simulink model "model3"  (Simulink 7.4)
settings: Solver=ode4  SolverMode=SingleTasking  StartTime=0.0  StopTime=10  FixedStep=1e-3  RelTol=1e-3
libraries: simulink x2

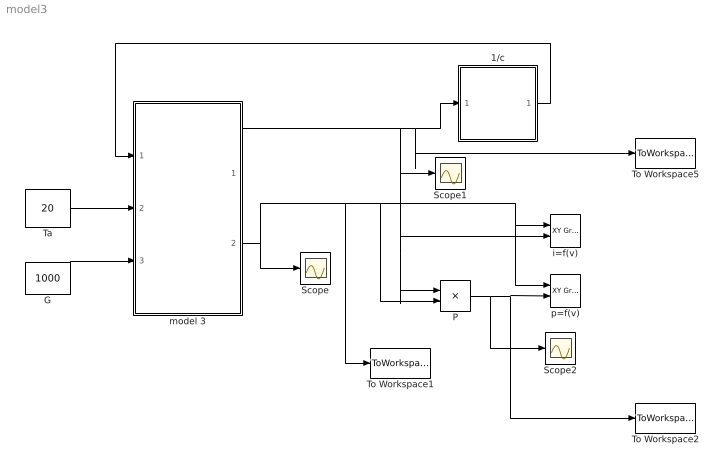
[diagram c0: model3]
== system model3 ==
  1/c : Subsystem
  G : Constant  Value=1000  OutDataType=sfix(16)  OutScaling=2^0
  P : Product  OutDataType=sfix(16)  OutScaling=2^0
  Scope : Scope
  Scope1 : Scope
  Scope2 : Scope
  Ta : Constant  Value=20  OutDataType=sfix(16)  OutScaling=2^0
  To Workspace1 : ToWorkspace  VariableName=v  SampleTime=-1  SaveFormat=Array
  To Workspace2 : ToWorkspace  VariableName=p  SampleTime=-1  SaveFormat=Array
  To Workspace5 : ToWorkspace  VariableName=i  SampleTime=-1  SaveFormat=Array
  i=f(v) : simulink/Sinks/XY Graph  SystemSampleTime=-1  xmin=0  xmax=50  ymin=0  ymax=5  st=-1
  model 3 : Subsystem  mask{beta_ref=-152e-3, alpha_ref=1.4e-3, Vm=35, Im=3.15, Voc=43.5, Isc=3.45, Tjref=25, Esref=1000, Noct=45}
  p=f(v) : simulink/Sinks/XY Graph  SystemSampleTime=-1  xmin=0  xmax=50  ymin=0  ymax=150  st=-1
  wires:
  1/c/1(Vdc) -> model 3/1(v)
  model 3/1(i+di) -> Scope1/1, P/1, i=f(v)/2, 1/c/1(Idc), To Workspace5/1
  P/1 -> Scope2/1, p=f(v)/2, To Workspace2/1
  model 3/2(v+dv1) -> Scope/1, i=f(v)/1, p=f(v)/1, P/2, To Workspace1/1
  Ta/1 -> model 3/2(Ta)
  G/1 -> model 3/3(G)

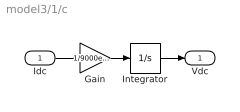
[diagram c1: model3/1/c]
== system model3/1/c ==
  Idc : Inport  OutDataType=sfix(16)  OutScaling=2^0
  Gain : Gain  Gain=1/9000e-5  ParameterDataType=sfix(16)  ParameterScaling=2^0  OutDataType=sfix(16)  OutScaling=2^0
  Integrator : Integrator
  Vdc : Outport
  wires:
  Gain/1 -> Integrator/1
  Integrator/1 -> Vdc/1
  Idc/1 -> Gain/1

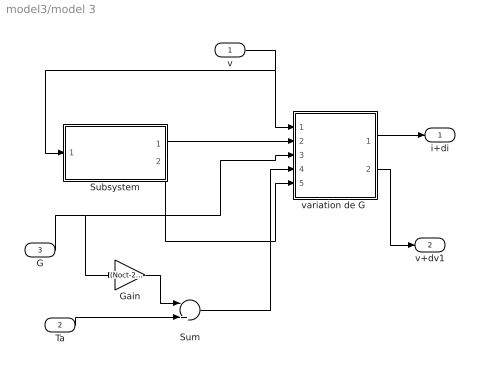
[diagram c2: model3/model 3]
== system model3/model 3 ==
  v : Inport  OutDataType=sfix(16)  OutScaling=2^0
  Ta : Inport  Port=2  OutDataType=sfix(16)  OutScaling=2^0
  G : Inport  Port=3  OutDataType=sfix(16)  OutScaling=2^0
  Gain : Gain  Gain=(Noct-20)/800  ParameterDataType=sfix(16)  ParameterScaling=2^0  OutDataType=sfix(16)  OutScaling=2^0
  Subsystem : Subsystem
  Sum : Sum  Inputs=|++  OutDataType=sfix(16)  OutScaling=2^0
  "variation de G " : Subsystem
  i+di : Outport
  v+dv1 : Outport  Port=2
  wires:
  Subsystem/1(I1) -> "variation de G "/2(I)
  G/1 -> "variation de G "/3(Es), Gain/1
  Subsystem/2(np) -> "variation de G "/5(np)
  "variation de G "/1(I+dI) -> i+di/1
  "variation de G "/2(V+dV) -> v+dv1/1
  v/1 -> "variation de G "/1(V), Subsystem/1(V)
  Ta/1 -> Sum/2
  Gain/1 -> Sum/1
  Sum/1 -> "variation de G "/4(Tj)

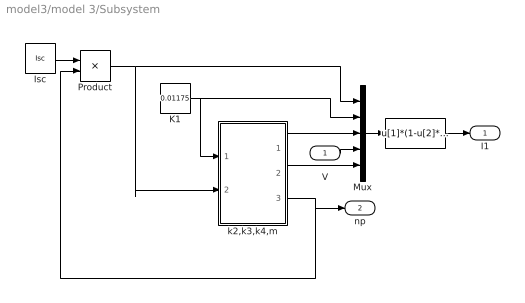
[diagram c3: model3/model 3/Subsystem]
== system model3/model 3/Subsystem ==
  V : Inport  OutDataType=sfix(16)  OutScaling=2^0
  I : Fcn  Expr=u[1]*(1-u[2]*(exp(u[3]*(u[4]^u[5]))-1))
  Isc : Constant  Value=Isc  OutDataType=sfix(16)  OutScaling=2^0
  K1 : Constant  Value=0.01175  OutDataType=sfix(16)  OutScaling=2^0
  Mux : Mux  Inputs=5
  Product : Product  OutDataType=sfix(16)  OutScaling=2^0
  k2,k3,k4,m : Subsystem
  I1 : Outport
  np : Outport  Port=2
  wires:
  Isc/1 -> Product/1
  K1/1 -> Mux/2, k2,k3,k4,m/1(k1)
  k2,k3,k4,m/1(k2) -> Mux/3
  k2,k3,k4,m/2(m) -> Mux/5
  Mux/1 -> I/1
  V/1 -> Mux/4
  I/1 -> I1/1
  k2,k3,k4,m/3(Np1) -> np/1, Product/2
  Product/1 -> Mux/1, k2,k3,k4,m/2(Isc)

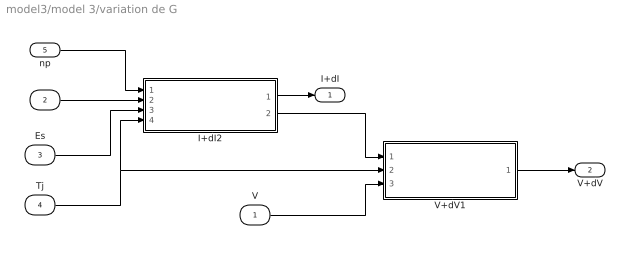
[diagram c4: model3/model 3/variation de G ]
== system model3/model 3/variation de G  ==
  V : Inport  OutDataType=sfix(16)  OutScaling=2^0
  I : Inport  Port=2  OutDataType=sfix(16)  OutScaling=2^0
  Es : Inport  Port=3  OutDataType=sfix(16)  OutScaling=2^0
  Tj : Inport  Port=4  OutDataType=sfix(16)  OutScaling=2^0
  np : Inport  Port=5  OutDataType=sfix(16)  OutScaling=2^0
  I+dI2 : Subsystem
  V+dV1 : Subsystem
  I+dI : Outport
  V+dV : Outport  Port=2
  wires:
  I/1 -> I+dI2/2(I)
  I+dI2/1(I+dI1) -> I+dI/1
  V/1 -> V+dV1/3(v)
  I+dI2/2(dI) -> V+dV1/1(dI)
  Tj/1 -> I+dI2/4(Tj), V+dV1/2(Tj)
  np/1 -> I+dI2/1(np)
  Es/1 -> I+dI2/3(Es)
  V+dV1/1(V+dV1) -> V+dV/1

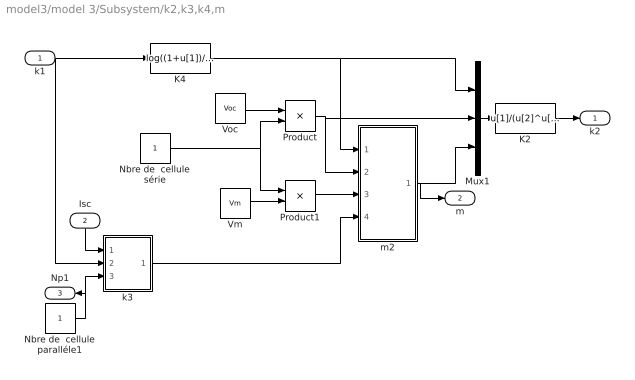
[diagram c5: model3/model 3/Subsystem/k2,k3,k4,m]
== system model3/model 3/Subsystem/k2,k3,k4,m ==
  k1 : Inport  OutDataType=sfix(16)  OutScaling=2^0
  Isc : Inport  Port=2  OutDataType=sfix(16)  OutScaling=2^0
  K2 : Fcn  Expr=u[1]/(u[2]^u[3])
  K4 : Fcn  Expr=log((1+u[1])/u[1])
  Mux1 : Mux  Inputs=3
  Nbre de  cellule paralléle1 : Constant  OutDataType=sfix(16)  OutScaling=2^0
  Nbre de  cellule série : Constant  OutDataType=sfix(16)  OutScaling=2^0
  Product : Product  OutDataType=sfix(16)  OutScaling=2^0
  Product1 : Product  OutDataType=sfix(16)  OutScaling=2^0
  Vm : Constant  Value=Vm  OutDataType=sfix(16)  OutScaling=2^0
  Voc : Constant  Value=Voc  OutDataType=sfix(16)  OutScaling=2^0
  k3 : Subsystem
  m2 : Subsystem
  k2 : Outport
  m : Outport  Port=2
  Np1 : Outport  Port=3
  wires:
  K4/1 -> Mux1/1, m2/1(k4)
  k1/1 -> K4/1, k3/2(k1)
  m2/1(m) -> Mux1/3, m/1
  Voc/1 -> Product/1
  Nbre de  cellule série/1 -> Product/2, Product1/1
  Product/1 -> Mux1/2, m2/2(Voc)
  Product1/1 -> m2/3(Vm)
  Vm/1 -> Product1/2
  Isc/1 -> k3/1(Isc)
  k3/1(k3) -> m2/4("k3 ")
  Nbre de  cellule paralléle1/1 -> k3/3(Np), Np1/1
  Mux1/1 -> K2/1
  K2/1 -> k2/1

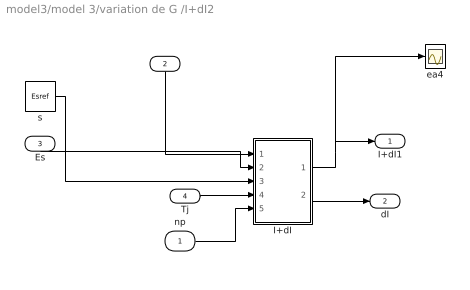
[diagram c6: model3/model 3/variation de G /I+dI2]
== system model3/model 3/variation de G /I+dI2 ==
  np : Inport  OutDataType=sfix(16)  OutScaling=2^0
  I : Inport  Port=2  OutDataType=sfix(16)  OutScaling=2^0
  Es : Inport  Port=3  OutDataType=sfix(16)  OutScaling=2^0
  Tj : Inport  Port=4  OutDataType=sfix(16)  OutScaling=2^0
  I+dI : Subsystem
  ea4 : Scope
  s : Constant  Value=Esref  OutDataType=sfix(16)  OutScaling=2^0
  I+dI1 : Outport
  dI : Outport  Port=2
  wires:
  Tj/1 -> I+dI/4(Tj)
  np/1 -> I+dI/5(np)
  s/1 -> I+dI/3(Esref)
  Es/1 -> I+dI/2(Es)
  I/1 -> I+dI/1(I)
  I+dI/2(dI1) -> dI/1
  I+dI/1(I+dI) -> ea4/1, I+dI1/1

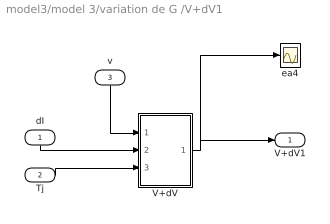
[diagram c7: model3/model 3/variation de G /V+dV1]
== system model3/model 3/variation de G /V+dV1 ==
  dI : Inport  OutDataType=sfix(16)  OutScaling=2^0
  Tj : Inport  Port=2  OutDataType=sfix(16)  OutScaling=2^0
  v : Inport  Port=3  OutDataType=sfix(16)  OutScaling=2^0
  V+dV : Subsystem
  ea4 : Scope
  V+dV1 : Outport
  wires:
  dI/1 -> V+dV/2(dI)
  Tj/1 -> V+dV/3(Tj)
  v/1 -> V+dV/1(V)
  V+dV/1(V+dV) -> ea4/1, V+dV1/1

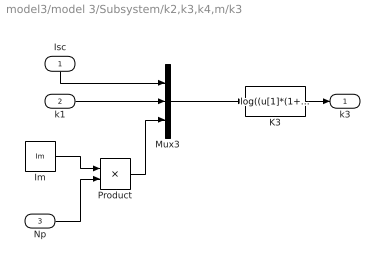
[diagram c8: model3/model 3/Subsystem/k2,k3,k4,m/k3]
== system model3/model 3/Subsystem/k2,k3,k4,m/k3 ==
  Isc : Inport  OutDataType=sfix(16)  OutScaling=2^0
  k1 : Inport  Port=2  OutDataType=sfix(16)  OutScaling=2^0
  Np : Inport  Port=3  OutDataType=sfix(16)  OutScaling=2^0
  Im : Constant  Value=Im  OutDataType=sfix(16)  OutScaling=2^0
  K3 : Fcn  Expr=log((u[1]*(1+u[2])-u[3])/(u[2]*u[1]))
  Mux3 : Mux  Inputs=3
  Product : Product  OutDataType=sfix(16)  OutScaling=2^0
  k3 : Outport
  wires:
  Isc/1 -> Mux3/1
  k1/1 -> Mux3/2
  Np/1 -> Product/2
  Im/1 -> Product/1
  Mux3/1 -> K3/1
  K3/1 -> k3/1
  Product/1 -> Mux3/3

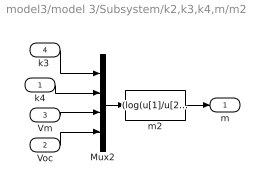
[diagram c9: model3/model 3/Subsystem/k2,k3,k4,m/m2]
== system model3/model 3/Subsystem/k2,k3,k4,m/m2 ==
  k4 : Inport  OutDataType=sfix(16)  OutScaling=2^0
  Voc : Inport  Port=2  OutDataType=sfix(16)  OutScaling=2^0
  Vm : Inport  Port=3  OutDataType=sfix(16)  OutScaling=2^0
  "k3 " : Inport  Port=4  OutDataType=sfix(16)  OutScaling=2^0
  Mux2 : Mux
  m2 : Fcn  Expr=(log(u[1]/u[2]))/(log(u[3]/u[4]))
  m : Outport
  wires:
  Mux2/1 -> m2/1
  k4/1 -> Mux2/2
  Voc/1 -> Mux2/4
  "k3 "/1 -> Mux2/1
  m2/1 -> m/1
  Vm/1 -> Mux2/3

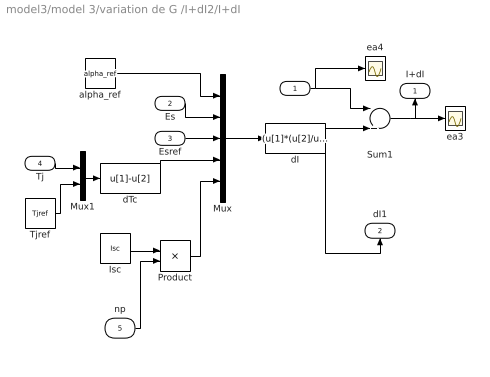
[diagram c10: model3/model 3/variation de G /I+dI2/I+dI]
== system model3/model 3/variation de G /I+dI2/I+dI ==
  I : Inport  OutDataType=sfix(16)  OutScaling=2^0
  Es : Inport  Port=2  OutDataType=sfix(16)  OutScaling=2^0
  Esref : Inport  Port=3  OutDataType=sfix(16)  OutScaling=2^0
  Tj : Inport  Port=4  OutDataType=sfix(16)  OutScaling=2^0
  np : Inport  Port=5  OutDataType=sfix(16)  OutScaling=2^0
  Isc : Constant  Value=Isc  OutDataType=sfix(16)  OutScaling=2^0
  Mux : Mux  Inputs=5
  Mux1 : Mux  Inputs=2
  Product : Product  OutDataType=sfix(16)  OutScaling=2^0
  Sum1 : Sum  Inputs=|++  OutDataType=sfix(16)  OutScaling=2^0
  Tjref : Constant  Value=Tjref  OutDataType=sfix(16)  OutScaling=2^0
  alpha_ref : Constant  Value=alpha_ref  OutDataType=sfix(16)  OutScaling=2^0
  dI : Fcn  Expr=(u[1]*(u[2]/u[3])*u[4])+(((u[2]/u[3])-1)*u[5])
  dTc : Fcn  Expr=u[1]-u[2]
  ea3 : Scope
  ea4 : Scope
  I+dI : Outport
  dI1 : Outport  Port=2
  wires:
  Mux/1 -> dI/1
  alpha_ref/1 -> Mux/1
  Esref/1 -> Mux/3
  dTc/1 -> Mux/4
  Es/1 -> Mux/2
  Sum1/1 -> ea3/1, I+dI/1
  Mux1/1 -> dTc/1
  Tjref/1 -> Mux1/2
  Tj/1 -> Mux1/1
  I/1 -> Sum1/1, ea4/1
  np/1 -> Product/2
  Isc/1 -> Product/1
  Product/1 -> Mux/5
  dI/1 -> Sum1/2, dI1/1

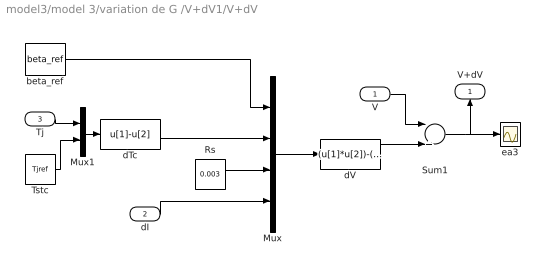
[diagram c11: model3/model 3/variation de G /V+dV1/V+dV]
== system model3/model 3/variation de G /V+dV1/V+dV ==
  V : Inport  OutDataType=sfix(16)  OutScaling=2^0
  dI : Inport  Port=2  OutDataType=sfix(16)  OutScaling=2^0
  Tj : Inport  Port=3  OutDataType=sfix(16)  OutScaling=2^0
  Mux : Mux
  Mux1 : Mux  Inputs=2
  Rs : Constant  Value=0.003  OutDataType=sfix(16)  OutScaling=2^0
  Sum1 : Sum  Inputs=|++  OutDataType=sfix(16)  OutScaling=2^0
  Tstc : Constant  Value=Tjref  OutDataType=sfix(16)  OutScaling=2^0
  beta_ref : Constant  Value=beta_ref  OutDataType=sfix(16)  OutScaling=2^0
  dTc : Fcn  Expr=u[1]-u[2]
  dV : Fcn  Expr=(u[1]*u[2])-(u[3]*u[4])
  ea3 : Scope
  V+dV : Outport
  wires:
  beta_ref/1 -> Mux/1
  Mux/1 -> dV/1
  dTc/1 -> Mux/2
  Rs/1 -> Mux/3
  dI/1 -> Mux/4
  Tj/1 -> Mux1/1
  Tstc/1 -> Mux1/2
  Mux1/1 -> dTc/1
  Sum1/1 -> V+dV/1, ea3/1
  V/1 -> Sum1/1
  dV/1 -> Sum1/2
